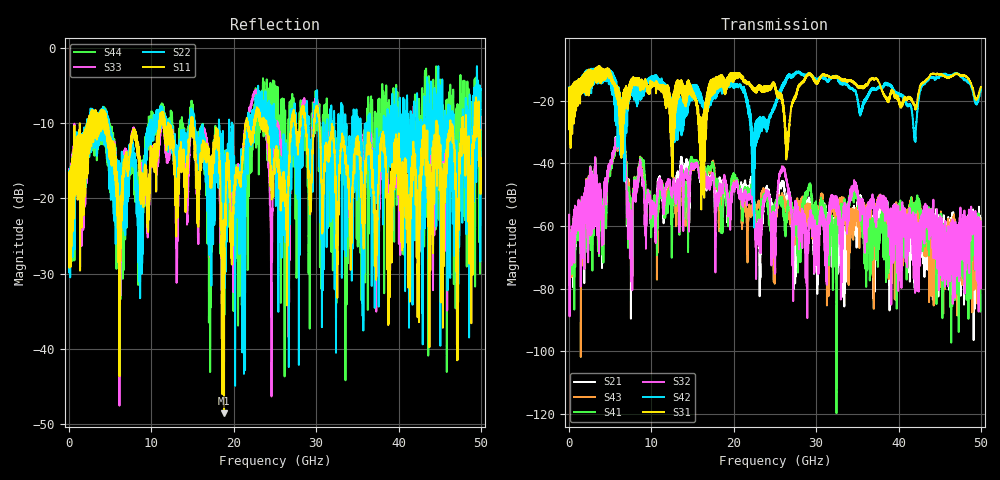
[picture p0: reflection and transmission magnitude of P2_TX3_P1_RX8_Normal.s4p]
!Keysight Technologies,N5225B,MY57041031,A.13.20.10
!Date: Friday, May 31, 2019 11:26:42
!Correction: S11(Full 4 Port(1,2,3,4))
!S12(Full 4 Port(1,2,3,4))
!S13(Full 4 Port(1,2,3,4))
!S14(Full 4 Port(1,2,3,4))
!S21(Full 4 Port(1,2,3,4))
!S22(Full 4 Port(1,2,3,4))
!S23(Full 4 Port(1,2,3,4))
!S24(Full 4 Port(1,2,3,4))
!S31(Full 4 Port(1,2,3,4))
!S32(Full 4 Port(1,2,3,4))
!S33(Full 4 Port(1,2,3,4))
!S34(Full 4 Port(1,2,3,4))
!S41(Full 4 Port(1,2,3,4))
!S42(Full 4 Port(1,2,3,4))
!S43(Full 4 Port(1,2,3,4))
!S44(Full 4 Port(1,2,3,4))
!S4P File: Measurements: <S11,S12,S13,S14>,
!<S21,S22,S23,S24>,
!<S31,S32,S33,S34>,
!<S41,S42,S43,S44>:
# Hz S  dB  R 50.0
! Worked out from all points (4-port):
!   5000 points, 10 MHz to 50 GHz, reference 50 ohm
!   strongest paths, dB at 10 MHz, 12.51 GHz, 25.01 GHz, 37.51 GHz, 50 GHz:
!     S31: -19.6, -43.2, -16.0, -13.6, -15.7
!     S42: -19.4, -24.3, -22.0, -16.0, -16.5
!     S32: -56.4, -50.4, -75.2, -52.9, -63.8
!     S41: -70.6, -65.6, -53.7, -57.8, -66.0
!     S43: -61.4, -54.3, -68.2, -53.3, -64.5
!     S21: -56.6, -55.4, -54.3, -54.5, -65.9
!   lowest |S11| = -48.6 dB at 18.82 GHz (marker M1), VSWR 1.01, Z = 49.6 + j0.0898 ohm
!   |S11| at or under -10 dB: 4.63 GHz to 10.95 GHz (6.318 GHz wide, 81.1 % of centre); 15.04 GHz to 21.46 GHz (6.426 GHz wide, 35.2 % of centre); 30.38 GHz to 44.6 GHz (14.22 GHz wide, 37.9 % of centre)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
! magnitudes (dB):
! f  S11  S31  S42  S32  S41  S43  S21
! 10 MHz  -19.5  -19.6  -19.4  -56.4  -70.6  -61.4  -56.6
! 5.85 GHz  -17.7  -19.2  -27.7  -34.6  -34.4  -35.1  -33.9
! 7.45 GHz  -13.5  -17.5  -17.4  -54.9  -50.7  -51.2  -52.4
! 18.82 GHz  -48.6  -13.3  -16.2  -45.2  -45.5  -45.4  -48.2
! 22.38 GHz  -11.2  -16.4  -39.4  -53.8  -48.9  -54.7  -49.3
! 27.71 GHz  -11.9  -16.9  -10.8  -53.9  -66.3  -51.6  -56.4
! 50 GHz  -15.7  -15.7  -16.5  -63.8  -66.0  -64.5  -65.9
